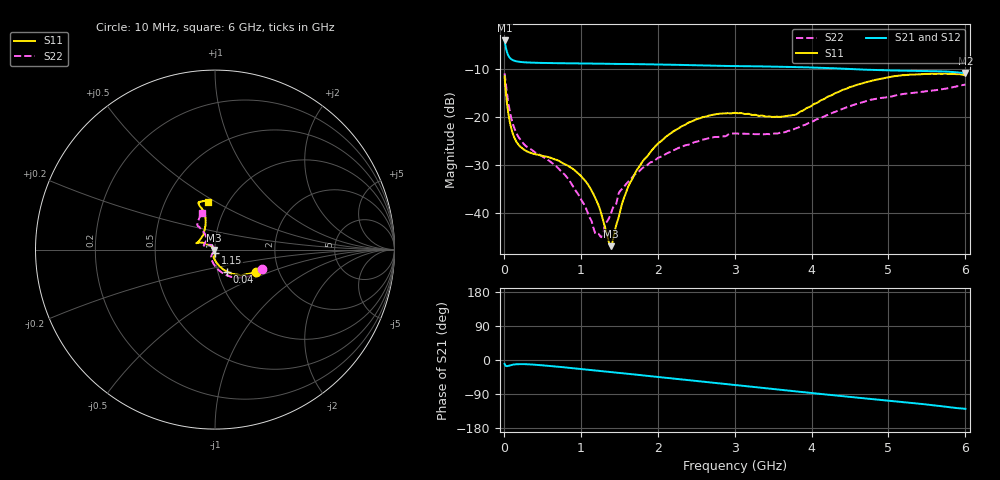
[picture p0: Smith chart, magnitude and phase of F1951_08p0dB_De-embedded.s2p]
! Integrated Device Technology
! Corporate Headquarters
! 6024 Silver Creek Valley Road
! San Jose, CA 95138  USA
! Phone:  1-408-284-8200
! Toll Free:  1-800-223-1366
! Webpage:  http://www.idt.com/
! Timing and RF Division
! 515 Groton Road, Suite 102
! Westford, MA 01886-6024
! Device:  F1951
! Description: 6-bit 0.5 dB Digital Step Attenuator
! Frequency:  100.0 -  4000.00 MHz
! Package:  4x4 mm Thin QFN Plastic Package: 24 pin
! Ports:  2 RF, 6 DC
!  Pin  1  = NC
!  Pin  2  = RF1  =  Port 1
!  Pin  3  = GND
!  Pin  4  = NC
!  Pin  5  = Serial Data Out (SDO)
!  Pin  6  = NC
!  Pin  7  = Reset Bar ( RSTb)
!  Pin  8  = Clock (CLK)
!  Pin  9  = Chip Select Bar (CSb)
!  Pin 10  = NC
!  Pin 11  = Serial Data In (SDI)
!  Pin 12  = NC
!  Pin 13  = NC
!  Pin 14  = VDD
!  Pin 15  = NC
!  Pin 16  = GND
!  Pin 17  = RF2  =  Port 2
!  Pin 18  = NC
!  Pin 19  = GND
!  Pin 20  = GND
!  Pin 21  = GND
!  Pin 22  = GND
!  Pin 23  = GND
!  Pin 24  = GND
! State:  16
! Atten State:  8.0 dB
! Voltage:  +3.30 Volts
! Current:  0.473 mA
! Data:  The device was measured on a F195X evaluation board which has
!  individual transmission lines to the RF pins.  Data was collected
!  de-embedded using a Automatic Fixture Removal [AFR] (Keysight Technologies).
!  The reference plane is the edge of the package pin.
! Misc:  Lot Code  1225BCA
!  Action Tracker AT0399
! Date Measured:  2018-09-13
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# GHz S dB R 50
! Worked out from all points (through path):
!   600 points, 10 MHz to 6 GHz, reference 50 ohm
!   highest |S21| = -4.18 dB at 10 MHz (marker M1); lowest = -10.9 dB at 6 GHz (marker M2)
!   group delay of S21, straight-line fit = 57.2 ps
!   lowest |S11| = -46.8 dB at 1.39 GHz (marker M3), VSWR 1.01, Z = 49.6 - j0.199 ohm
!   |S11| at or under -10 dB: start of sweep to end of sweep
!   |S22| runs from -44.9 to -11.0 dB; largest |S21 - S12| = 0.00056
!   S11 on the Smith chart (normalised r, x): 10 MHz: 1.53, -0.42; 40 MHz: 1.11, -0.28; 1.15 GHz: 1.00, -0.03; 6 GHz: 0.80, +0.46
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0.01  -11.64 -28.9  -4.18 -10.4  -4.18 -10.4  -10.99 -23.0
0.04  -17.11 -61.5  -6.54 -16.2  -6.53 -16.3  -15.03 -59.0
0.07  -20.40 -74.9  -7.61 -14.7  -7.61 -14.7  -18.25 -77.3
0.11  -23.17 -84.8  -8.20 -12.5  -8.20 -12.5  -21.07 -91.3
0.21  -26.11 -97.0  -8.62 -10.8  -8.62 -10.9  -24.61 -109.1
0.77  -29.65 -93.8  -8.90 -19.0  -8.90 -19.1  -31.65 -120.8
1.01  -32.38 -87.2  -8.96 -23.8  -8.96 -23.8  -37.30 -121.5
1.15  -35.55 -88.4  -8.98 -26.6  -8.98 -26.6  -42.10 -140.3
1.2  -37.18 -90.8  -8.98 -27.6  -8.99 -27.6  -44.30 -159.9
1.26  -39.72 -95.6  -8.99 -28.9  -9.00 -28.9  -44.86 174.4
1.39  -46.79 -154.0  -9.02 -31.6  -9.02 -31.6  -40.07 131.0
1.51  -39.67 147.5  -9.04 -34.1  -9.05 -34.1  -35.40 124.0
1.63  -33.98 140.2  -9.06 -36.7  -9.06 -36.7  -33.23 121.2
1.8  -29.32 139.6  -9.10 -40.4  -9.10 -40.4  -30.64 124.9
2.01  -25.46 144.7  -9.16 -44.9  -9.16 -44.9  -28.45 133.0
2.49  -20.57 155.1  -9.31 -55.2  -9.31 -55.2  -25.19 150.7
3.01  -19.19 161.2  -9.48 -66.2  -9.48 -66.1  -23.43 157.7
3.6  -20.01 139.6  -9.61 -78.6  -9.62 -78.6  -23.22 138.5
4.01  -17.59 114.8  -9.78 -87.3  -9.78 -87.3  -21.01 124.7
4.5  -13.84 106.2  -10.09 -97.4  -10.09 -97.4  -17.79 123.5
5.01  -11.80 109.4  -10.39 -107.2  -10.39 -107.2  -15.91 125.9
6  -11.35 98.5  -10.94 -128.8  -10.94 -128.8  -13.30 110.2
